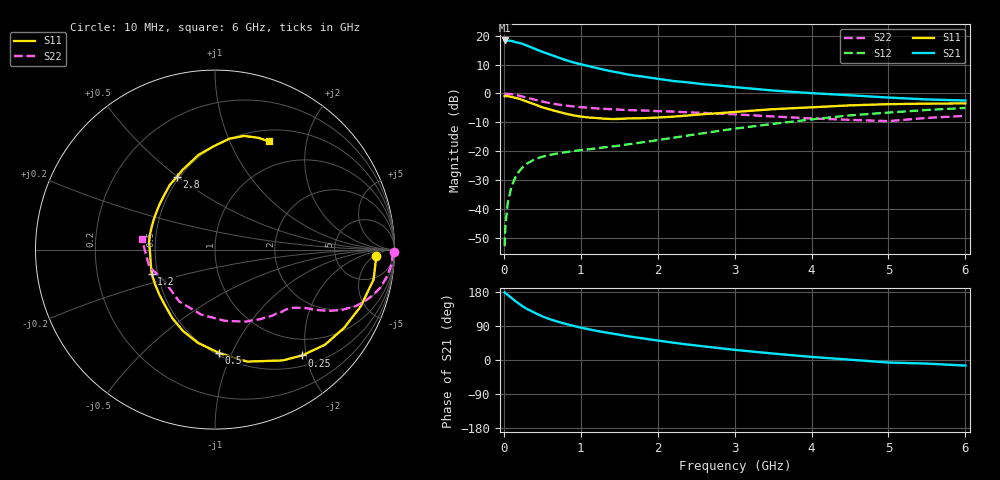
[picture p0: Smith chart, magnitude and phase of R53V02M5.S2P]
! SIEMENS Small Signal Semiconductors
! BFR183
! Si NPN RF Bipolar Junction Transistor in SOT23
! VCE = 3 V  IC = 2.5 mA
! Common Emitter S-Parameters:  May  1996
# GHz  S  MA  R  50
!  f  S11  S21  S12  S22
! GHz  MAG  ANG  MAG  ANG  MAG  ANG  MAG  ANG
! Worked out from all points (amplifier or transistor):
!   36 points, 10 MHz to 6 GHz, reference 50 ohm
!   highest |S21| = 18.3 dB at 10 MHz (marker M1)
!   |S21| within 3 dB of that: start of sweep to 413 MHz
!   unconditionally stable (mu >= 1): 1.307 GHz to 2.795 GHz
!   at 250 MHz: K = 0.26, MSG = 21.2 dB, |S12| = -25.3 dB
!   at 1.4 GHz: K = 1.04, MAG = 11.8 dB, |S12| = -18.3 dB
!   at 6 GHz: K = 0.90, MSG = 1.3 dB, |S12| = -5.0 dB
!   S11 on the Smith chart (normalised r, x): 10 MHz: 17, -6; 250 MHz: 0.68, -1.93; 500 MHz: 0.52, -0.90; 1.2 GHz: 0.46, -0.14; 2.8 GHz: 0.48, +0.50; 6 GHz: 0.64, +1.41
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0.01  0.9003 -2.1  8.252 178.6  0.0023 86.9  0.995 -0.9
0.02  0.8976 -4.5  8.15 176.6  0.005 88.2  0.989 -1.7
0.05  0.8992 -10.7  8.151 171.8  0.0127 83.7  0.9889 -4.5
0.1  0.8714 -21.3  8.122 163.7  0.0249 79.6  0.9701 -8.7
0.15  0.8414 -31.1  7.73 155.2  0.0355 72.6  0.9469 -12.8
0.25  0.764 -50.5  7.166 140.9  0.0541 63.9  0.8799 -19.3
0.3  0.7241 -58.5  6.715 134.7  0.0613 60.7  0.8459 -21.8
0.4  0.6492 -74.0  5.936 124.8  0.0729 54.8  0.7832 -25.4
0.5  0.5766 -87.7  5.25 115.1  0.0809 50.6  0.727 -28.0
0.6  0.5281 -100.4  4.715 107.6  0.087 48.4  0.6808 -29.8
0.7  0.4868 -111.6  4.224 101.2  0.092 46.9  0.6463 -31.2
0.8  0.4505 -121.7  3.795 95.5  0.0966 45.8  0.6181 -32.1
0.9  0.4197 -131.0  3.459 90.3  0.1013 45.5  0.5988 -32.9
1.1  0.3852 -150.4  2.977 81.3  0.1084 46.5  0.5668 -34.9
1.2  0.377 -159.2  2.769 77.1  0.1125 47.1  0.5535 -35.8
1.6  0.3701 173.2  2.146 63.1  0.1314 50.4  0.5181 -40.1
2.2  0.3978 141.3  1.647 45.8  0.1716 54.1  0.4873 -49.2
2.8  0.4568 117.7  1.369 31.4  0.2259 53.8  0.4474 -61.6
3.5  0.536 99.8  1.126 17.0  0.2983 48.9  0.4007 -82.2
4.5  0.6237 82.5  0.931 0.8  0.419 37.1  0.3508 -124.8
5.5  0.6679 68.8  0.789 -9.5  0.5192 23.1  0.3786 -165.4
6  0.6739 63.5  0.756 -14.7  0.563 14.2  0.411 172.0
